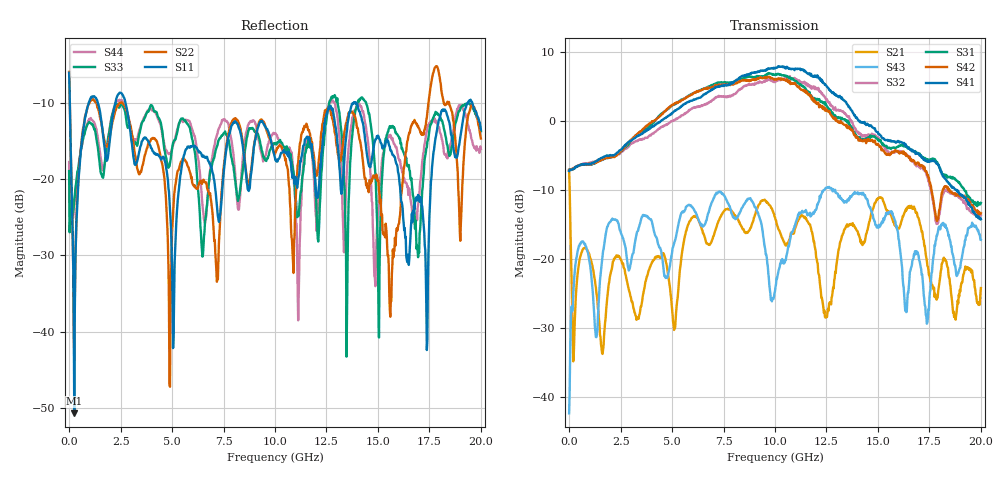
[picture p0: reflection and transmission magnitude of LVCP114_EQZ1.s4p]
!Agilent Technologies,N5230A,MY46400459,A.07.50.48
!Agilent N5230A: A.07.50.48
!Date: Monday, January 09, 2012 14:02:08
!Correction: S11(Full 4 Port(1,2,3,4))
!S12(Full 4 Port(1,2,3,4))
!S13(Full 4 Port(1,2,3,4))
!S14(Full 4 Port(1,2,3,4))
!S21(Full 4 Port(1,2,3,4))
!S22(Full 4 Port(1,2,3,4))
!S23(Full 4 Port(1,2,3,4))
!S24(Full 4 Port(1,2,3,4))
!S31(Full 4 Port(1,2,3,4))
!S32(Full 4 Port(1,2,3,4))
!S33(Full 4 Port(1,2,3,4))
!S34(Full 4 Port(1,2,3,4))
!S41(Full 4 Port(1,2,3,4))
!S42(Full 4 Port(1,2,3,4))
!S43(Full 4 Port(1,2,3,4))
!S44(Full 4 Port(1,2,3,4))
!S4P File: Measurements: <S11,S12,S13,S14>,
!<S21,S22,S23,S24>,
!<S31,S32,S33,S34>,
!<S41,S42,S43,S44>:
# Hz S  dB  R 50
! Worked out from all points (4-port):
!   801 points, 300 kHz to 20 GHz, reference 50 ohm
!   strongest paths, dB at 300 kHz, 5 GHz, 10 GHz, 15 GHz, 20 GHz:
!     S41: -7.2, 1.1, 7.7, -1.6, -14.2
!     S42: -7.1, 2.3, 6.0, -3.3, -13.3
!     S31: -7.2, 2.2, 6.7, -2.8, -11.9
!     S32: -7.0, 0.0, 5.7, -2.5, -13.6
!     S43: -42.3, -19.1, -24.6, -15.3, -17.2
!     S21: -7.1, -27.1, -13.9, -11.1, -24.2
!   lowest |S11| = -50.7 dB at 250.3 MHz (marker M1), VSWR 1.01, Z = 50.2 - j0.169 ohm
!   |S11| at or under -10 dB: 34.42 MHz to 951.8 MHz (917.4 MHz wide, 186 % of centre); 2.738 GHz to 13.82 GHz (11.08 GHz wide, 134 % of centre); 13.95 GHz to 19.36 GHz (5.411 GHz wide, 32.5 % of centre)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
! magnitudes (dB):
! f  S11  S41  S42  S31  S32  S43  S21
! 300 kHz  -6.0  -7.2  -7.1  -7.2  -7.0  -42.3  -7.1
! 250.3 MHz  -50.7  -6.8  -6.8  -6.9  -6.8  -22.6  -31.1
! 1.15 GHz  -9.2  -6.1  -6.1  -6.2  -5.9  -24.8  -21.4
! 4.9 GHz  -24.0  1.0  2.1  2.1  -0.2  -20.9  -24.1
! 8 GHz  -12.5  5.6  5.3  5.7  3.9  -14.0  -13.4
! 15.6 GHz  -16.2  -2.9  -4.8  -4.0  -4.7  -13.2  -13.4
! 20 GHz  -13.5  -14.2  -13.3  -11.9  -13.6  -17.2  -24.2
